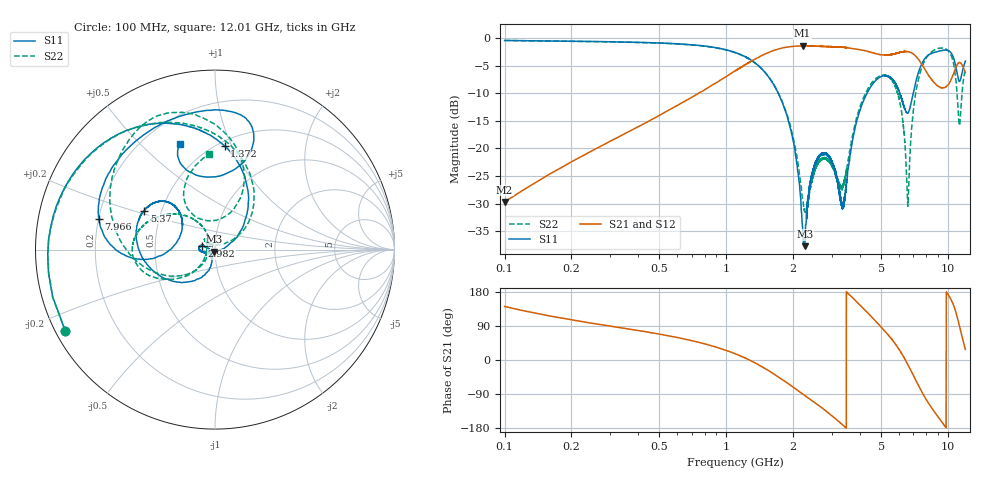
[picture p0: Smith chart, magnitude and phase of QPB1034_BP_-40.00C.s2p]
! TDS: k:\Engsetup\Winsaw\QPB1034_ALL
! Channel 1
! Ports=1 2
! seg 1=100.000000 1100.000000 51
! seg 2=1101.000000 1301.000000 201
! seg 3=1302.000000 2302.000000 101
! seg 4=2303.000000 3503.000000 1201
! seg 5=3504.000000 5204.000000 171
! seg 6=5205.000000 6405.000000 1201
! seg 7=6406.000000 8506.000000 211
! seg 8=8507.000000 12007.000000 176
! Points=3313
! FailCode=0
! Topology=ALL_SE(12)
!VNA Cal loaded =QPB1034_ALL_-40C
!PS1(V)= 5.000
!PS(mA)= 0.661
!PS2(V)= 1.170
!PS(mA)= -0.001
!PS3(V)= 1.170
!PS(mA)= 0.000
!PS4(V)= 1.170
!PS(mA)= -0.001
!Temp (C)= -40.00
# MHz S DB R 50
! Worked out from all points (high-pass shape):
!   3313 points, 100 MHz to 12.01 GHz, reference 50 ohm
!   highest |S21| = -1.42 dB at 2.212 GHz (marker M1); lowest = -29.7 dB at 100 MHz (marker M2)
!   |S21| within 3 dB of the highest: 1.26943 GHz to 1.270602 GHz (1.171 MHz wide, 0.0922 % of centre); 1.272 GHz to 7.536 GHz (6.264 GHz wide, 142 % of centre)
!   lowest |S11| = -37.7 dB at 2.262 GHz (marker M3), VSWR 1.03, Z = 49.5 - j1.2 ohm
!   |S11| at or under -10 dB: 1.715 GHz to 4.32 GHz (2.605 GHz wide, 86.3 % of centre); 6.0744 GHz to 6.077985 GHz (3.585 MHz wide, 0.059 % of centre); 6.078 GHz to 6.981 GHz (903.2 MHz wide, 13.8 % of centre)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
!   |S22| runs from -31.8 to -0.4 dB; largest |S21 - S12| = 0.007
!   S11 on the Smith chart (normalised r, x): 100 MHz: 0.03, -0.25; 1.372 GHz: 0.54, +0.94; 2.982 GHz: 0.86, +0.04; 5.37 GHz: 0.40, +0.22; 7.966 GHz: 0.20, +0.12; 12.01 GHz: 0.35, +0.66
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100  -0.45 -151.5  -29.70 141.2  -29.71 141.0  -0.45 -151.4
240  -0.63 179.1  -20.75 98.2  -20.74 98.3  -0.64 179.4
500  -0.91 154.6  -14.01 68.3  -14.01 68.2  -0.92 155.1
1100  -2.64 108.2  -5.91 16.4  -5.93 16.3  -2.67 106.0
1372  -4.75 84.7  -3.67 -9.8  -3.67 -10.0  -4.76 80.4
1842  -13.00 42.9  -1.71 -56.4  -1.71 -56.4  -12.80 38.0
2212  -34.27 -34.2  -1.42 -89.3  -1.45 -89.1  -29.12 53.3
2262  -37.70 -111.4  -1.42 -93.2  -1.43 -93.3  -31.69 80.7
2434  -24.75 -163.5  -1.47 -106.6  -1.44 -106.7  -26.06 137.3
2982  -22.46 163.8  -1.56 -145.8  -1.57 -145.8  -22.90 133.9
3371  -30.08 -147.3  -1.67 -172.5  -1.70 -172.4  -26.85 -170.3
4044  -12.74 -129.0  -2.14 143.7  -2.14 143.7  -12.13 -140.5
5370  -6.93 151.2  -3.06 66.9  -3.06 66.9  -6.99 170.2
5406  -6.95 149.6  -3.07 65.0  -3.04 64.9  -7.06 168.6
6113  -10.35 132.9  -2.57 22.5  -2.59 22.4  -12.13 130.6
6606  -13.62 162.0  -2.48 -11.9  -2.48 -12.0  -30.46 175.2
7136  -8.29 -172.0  -3.21 -50.8  -3.21 -50.8  -10.47 -150.8
7966  -3.49 165.2  -5.99 -102.9  -5.97 -103.1  -3.72 154.0
9347  -2.29 104.7  -9.00 -161.6  -8.98 -161.6  -1.82 114.3
10567  -3.39 71.4  -6.65 147.2  -6.65 147.5  -4.25 81.3
11287  -7.85 93.0  -4.43 89.6  -4.44 89.7  -15.85 96.7
12007  -4.18 108.5  -6.27 27.9  -6.28 28.0  -5.49 93.7
